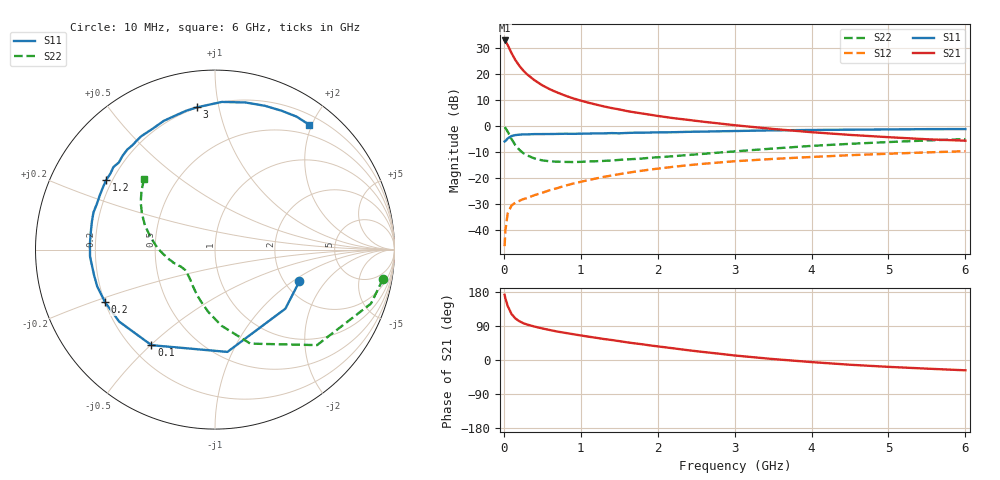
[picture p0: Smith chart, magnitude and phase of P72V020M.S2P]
! SIEMENS Small Signal Semiconductors
! BFP196
! Si NPN RF Bipolar Junction Transistor in SOT143
! VCE = 2 V  IC = 20 mA
! Common Emitter S-Parameters:  May  1996
# GHz  S  MA  R  50
!  f  S11  S21  S12  S22
! GHz  MAG  ANG  MAG  ANG  MAG  ANG  MAG  ANG
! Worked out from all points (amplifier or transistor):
!   36 points, 10 MHz to 6 GHz, reference 50 ohm
!   highest |S21| = 33.0 dB at 10 MHz (marker M1)
!   |S21| within 3 dB of that: start of sweep to 69.77 MHz
!   unconditionally stable (mu >= 1): 640.6 MHz to 3.445 GHz
!   at 250 MHz: K = 0.61, MSG = 24.9 dB, |S12| = -28.2 dB
!   at 1.4 GHz: K = 1.11, MAG = 11.0 dB, |S12| = -19.1 dB
!   at 6 GHz: K = 0.97, MSG = 2.0 dB, |S12| = -9.7 dB
!   S11 on the Smith chart (normalised r, x): 10 MHz: 2.39, -1.14; 100 MHz: 0.28, -0.50; 200 MHz: 0.20, -0.22; 1.2 GHz: 0.18, +0.28; 3 GHz: 0.20, +0.86; 6 GHz: 0.34, +1.96
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0.01  0.5023 -20.7  44.66 172.0  0.0048 85.6  0.9507 -9.9
0.02  0.512 -40.0  42.99 162.7  0.0096 76.3  0.9196 -19.1
0.05  0.5742 -83.1  36.4 142.4  0.0206 59.0  0.7788 -43.1
0.1  0.6394 -123.6  25.5 121.3  0.0293 45.8  0.5597 -69.4
0.15  0.6679 -143.1  18.7 109.7  0.0333 40.2  0.4258 -85.1
0.2  0.6791 -154.5  14.62 102.5  0.0358 39.7  0.3495 -96.1
0.25  0.6876 -162.6  11.84 97.4  0.0387 40.4  0.3004 -104.9
0.3  0.6887 -168.0  9.986 93.8  0.0406 41.7  0.2724 -111.5
0.4  0.6973 -176.8  7.605 88.1  0.0464 44.7  0.2355 -122.0
0.5  0.6979 177.4  6.09 83.3  0.0515 47.4  0.217 -129.4
0.6  0.699 171.7  5.094 79.0  0.0579 49.6  0.2081 -134.9
0.8  0.7082 163.0  3.841 71.5  0.0707 51.9  0.2027 -142.6
0.9  0.7057 158.9  3.414 68.1  0.0773 52.5  0.2014 -145.4
1.1  0.714 151.1  2.812 61.6  0.0903 52.6  0.2063 -149.6
1.2  0.7195 147.5  2.587 58.6  0.0973 52.6  0.209 -151.6
1.6  0.7336 134.6  1.942 46.7  0.1243 50.0  0.2271 -158.4
2.2  0.7579 117.2  1.42 30.9  0.163 43.7  0.2609 -167.8
3  0.7988 97.3  1.035 11.9  0.2086 33.8  0.3237 177.6
3.5  0.8238 87.3  0.876 2.5  0.2316 27.6  0.3672 168.8
4.5  0.8481 70.8  0.673 -12.5  0.2732 16.2  0.4525 154.0
5.5  0.8691 58.5  0.554 -22.8  0.3093 5.3  0.5254 141.2
6  0.8716 52.9  0.52 -27.2  0.3265 -0.5  0.5577 135.1
